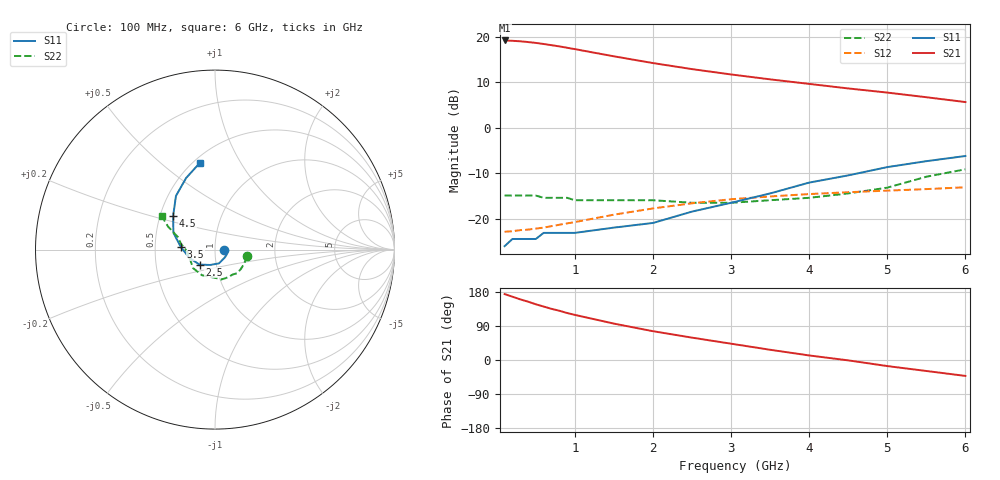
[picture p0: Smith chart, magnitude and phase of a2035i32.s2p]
!  MSA-2035 S AND NOISE PARAMETERS
!  Id = 32 mA  LAST UPDATED 06-27-94
# ghz s ma r 50
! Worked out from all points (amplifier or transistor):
!   20 points, 100 MHz to 6 GHz, reference 50 ohm
!   highest |S21| = 19.2 dB at 100 MHz (marker M1)
!   |S21| within 3 dB of that: start of sweep to 1.346 GHz
!   unconditionally stable (mu >= 1): start of sweep to 5.311 GHz
!   at 400 MHz: K = 1.07, MAG = 19.1 dB, |S12| = -22.4 dB
!   at 1.5 GHz: K = 1.04, MAG = 16.1 dB, |S12| = -19.1 dB
!   at 6 GHz: K = 0.91, MSG = 9.4 dB, |S12| = -13.1 dB
!   S11 on the Smith chart (normalised r, x): 100 MHz: 1.11, -0.00; 2.5 GHz: 0.83, -0.14; 3.5 GHz: 0.68, +0.02; 4.5 GHz: 0.58, +0.24; 6 GHz: 0.54, +0.68
0.1  0.05 -2.0  9.13 174.0  0.072 3.0  0.18 -11.0
0.2  0.06 -3.0  9.05 167.0  0.073 6.0  0.18 -20.0
0.3  0.06 -7.0  8.94 160.0  0.075 9.0  0.18 -29.0
0.4  0.06 -10.0  8.77 154.0  0.076 11.0  0.18 -38.0
0.5  0.06 -14.0  8.58 147.0  0.078 14.0  0.18 -47.0
0.6  0.07 -22.0  8.35 141.0  0.08 16.0  0.17 -55.0
0.7  0.07 -27.0  8.1 135.0  0.083 17.0  0.17 -63.0
0.8  0.07 -32.0  7.86 130.0  0.086 19.0  0.17 -71.0
0.9  0.07 -37.0  7.59 124.0  0.089 20.0  0.17 -79.0
1  0.07 -42.0  7.33 119.0  0.092 22.0  0.16 -86.0
1.5  0.08 -74.0  6.11 96.0  0.111 24.0  0.16 -117.0
2  0.09 -108.0  5.15 76.0  0.13 23.0  0.16 -140.0
2.5  0.12 -136.0  4.42 59.0  0.148 20.0  0.15 -155.0
3  0.15 -162.0  3.86 43.0  0.164 16.0  0.15 -169.0
3.5  0.19 176.0  3.41 27.0  0.176 11.0  0.16 -178.0
4  0.25 158.0  3.04 12.0  0.187 7.0  0.17 177.0
4.5  0.3 141.0  2.71 -1.0  0.196 3.0  0.19 171.0
5  0.37 126.0  2.44 -16.0  0.204 -1.0  0.22 161.0
5.5  0.43 112.0  2.17 -29.0  0.212 -5.0  0.29 154.0
6  0.49 100.0  1.92 -42.0  0.222 -9.0  0.35 148.0
